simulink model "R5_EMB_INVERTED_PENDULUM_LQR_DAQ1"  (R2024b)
settings: Solver=FixedStepDiscrete  StartTime=0.0  StopTime=S  FixedStep=T  RelTol=1e-3  EnableMultiTasking=on
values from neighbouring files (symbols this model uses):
  A_obs_d = Ad - Ld*C_meas    [R5_EMB_INVERTED_PENDULUM_LQR_DAQ1_script.m]
  B_obs_d = [Bd, Ld]    [R5_EMB_INVERTED_PENDULUM_LQR_DAQ1_script.m]
  C_obs_d = eye(4)    [R5_EMB_INVERTED_PENDULUM_LQR_DAQ1_script.m]
  D_obs_d = zeros(4, 1 + size(C_meas,1))    [R5_EMB_INVERTED_PENDULUM_LQR_DAQ1_script.m]
  Kd = dlqr(Ad, Bd, Q, R)    [R5_EMB_INVERTED_PENDULUM_LQR_DAQ1_script.m]
  Kt = Kt*motor_eff    (= 0.0273)    [R5_EMB_INVERTED_PENDULUM_LQR_DAQ1_script.m]
  r = 0.01    [R5_EMB_INVERTED_PENDULUM_LQR_DAQ1_script.m]
  T = 0.001    [R5_EMB_INVERTED_PENDULUM_LQR_DAQ1_script.m]
undefined symbols (not defined in the file or in its folder): Serial_Port, Standard_Devices
libraries: easyio x6, simulink x5

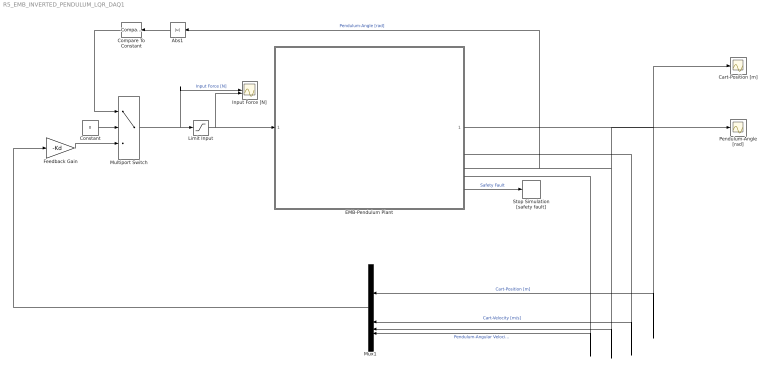
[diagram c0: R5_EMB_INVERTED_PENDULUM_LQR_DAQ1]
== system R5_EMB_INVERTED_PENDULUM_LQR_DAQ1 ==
  Abs1 : Abs
  Cart-Position [m] : Scope
  Compare To Constant : simulink/Logic and Bit Operations/Compare To Constant  relop=<=  const=0.2  OutDataTypeStr=boolean
  Constant : Constant  Value=0
  EMB-Pendulum Plant : Subsystem
  Feedback Gain : Gain  Gain=-Kd  Multiplication=Matrix(K*u)
  Input Force [N] : Scope  NumInputPorts=2
  Limit Input : Saturate  UpperLimit=10  LowerLimit=-10
  Multiport Switch : MultiPortSwitch  DataPortOrder=Zero-based contiguous  Inputs=2  zeroidx=on
  Mux1 : Mux
  Pendulum-Angle [rad] : Scope
  Stop Simulation [safety fault] : Stop
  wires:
  EMB-Pendulum Plant/5(Out5) -> Stop Simulation [safety fault]/1  "Safety Fault"
  Compare To Constant/1 -> Multiport Switch/1
  Multiport Switch/1 -> Input Force [N]/1, Limit Input/1  "Input Force [N]"
  Feedback Gain/1 -> Multiport Switch/3
  Abs1/1 -> Compare To Constant/1
  Limit Input/1 -> EMB-Pendulum Plant/1(In1), Input Force [N]/2
  Constant/1 -> Multiport Switch/2
  Mux1/1 -> Feedback Gain/1
  EMB-Pendulum Plant/4(Out4) -> Mux1/4  "Pendulum-Angular Velocity [rad/s]"
  EMB-Pendulum Plant/1(Out1) -> Cart-Position [m]/1, Mux1/1  "Cart-Position [m]"
  EMB-Pendulum Plant/3(Out3) -> Abs1/1, Mux1/3, Pendulum-Angle [rad]/1  "Pendulum-Angle [rad]"
  EMB-Pendulum Plant/2(Out2) -> Mux1/2  "Cart-Velocity [m/s]"

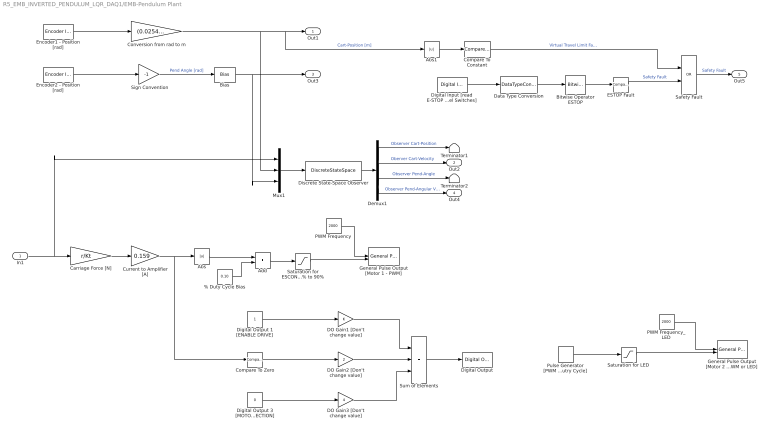
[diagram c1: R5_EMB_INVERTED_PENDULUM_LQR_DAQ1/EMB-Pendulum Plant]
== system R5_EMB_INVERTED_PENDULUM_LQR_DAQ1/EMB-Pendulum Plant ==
  In1 : Inport
  " Sign Convention" : Gain  Gain=-1
  % Duty Cycle Bias : Constant  Value=0.10  SampleTime=T
  Abs : Abs
  Abs1 : Abs
  Add : Sum
  Bias : Bias  Bias=-pi
  Bitwise Operator ESTOP : simulink/Logic and Bit Operations/Bitwise Operator  logicop=AND  UseBitMask=on  BitMask=8  BitMaskRealWorld=Real World Value
  Carriage Force [N] : Gain  Gain=r/Kt
  Compare To Constant : simulink/Logic and Bit Operations/Compare To Constant  relop=>=  const=0.035  OutDataTypeStr=boolean
  Compare To Zero : simulink/Logic and Bit Operations/Compare To Zero  relop=>=  OutDataTypeStr=boolean
  Conversion from rad to m : Gain  Gain=(0.0254)/(2*pi)
  Current to Amplifier [A] : Gain  Gain=0.159
  DO Gain1 [Don't change value] : Gain
  DO Gain2 [Don't change value] : Gain  Gain=2
  DO Gain3 [Don't change value] : Gain  Gain=4
  Data Type Conversion : DataTypeConversion  OutDataTypeStr=uint8  RndMeth=Nearest
  Demux1 : Demux
  Digital Input [read E-STOP and End of Travel Switches] : easyio/Digital Input  SampleTime=T  MaxMissedTicks=10  ShowMissedTicks=0  YieldWhenWaiting=0  DrvName=Standard_Devices/Serial_Port  DrvAddress=6  DrvOptions=[460800 8 0 0 0 0 0 0]  PacketSize=8  DataTypes='double'  ShowReady=0  ShowError=0  PacketID=1  ByteOrder=1  ShowTimestamp=0  CfgPrm=D0  PrmCfg=18  ResVar=0  VarRes=0  d7=off  d6=off  d5=off  d4=on  d3=on  d2=off  d1=off  d0=off
  Digital Output : easyio/Digital Output  SampleTime=T  MaxMissedTicks=10  ShowMissedTicks=0  YieldWhenWaiting=0  DrvName=Standard_Devices/Serial_Port  DrvAddress=6  DrvOptions=[460800 8 0 0 0 0 0 0]  PacketSize=8  DataTypes='double'  ShowReady=0  ShowError=0  PacketID=1  ByteOrder=1  InitialValue=0  FinalValue=0  CfgPrm=G0  PrmCfg=F8  ResVar=0  VarRes=0  d7=off  d6=off  d5=off  d4=off  d3=off  d2=on  d1=on  d0=on
  Digital Output 1 [ENABLE DRIVE] : Constant  SampleTime=T
  Digital Output 3 [MOTOR 2 DIRECTION] : Constant  Value=0  SampleTime=T
  Discrete State-Space Observer : DiscreteStateSpace  A=A_obs_d  B=B_obs_d  C=C_obs_d  D=D_obs_d  InitialCondition=[0 0 0 0]  SampleTime=T
  ESTOP Fault : simulink/Logic and Bit Operations/Compare To Constant  relop=~=  const=8  OutDataTypeStr=boolean
  Encoder1 - Position [rad] : easyio/Encoder Input  SampleTime=T  MaxMissedTicks=10  ShowMissedTicks=0  YieldWhenWaiting=0  DrvName=Standard_Devices/Serial_Port  DrvAddress=6  DrvOptions=[460800 8 0 0 0 0 0 0]  PacketSize=8  DataTypes='double'  ShowReady=0  ShowError=0  PacketID=1  ByteOrder=1  ShowTimestamp=0  CfgPrm=E0  PrmCfg=position  ResVar=0  VarRes=2000
  Encoder2 - Position [rad] : easyio/Encoder Input  SampleTime=T  MaxMissedTicks=10  ShowMissedTicks=0  YieldWhenWaiting=0  DrvName=Standard_Devices/Serial_Port  DrvAddress=6  DrvOptions=[460800 8 0 0 0 0 0 0]  PacketSize=8  DataTypes='double'  ShowReady=0  ShowError=0  PacketID=1  ByteOrder=1  ShowTimestamp=0  CfgPrm=E1  PrmCfg=position  ResVar=0  VarRes=2048
  General Pulse Output [Motor 1 - PWM] : easyio/General Pulse Output  SampleTime=T  MaxMissedTicks=10  ShowMissedTicks=0  YieldWhenWaiting=0  DrvName=Standard_Devices/Serial_Port  DrvAddress=6  DrvOptions=[460800 8 0 0 0 0 0 0]  PacketSize=16  DataTypes={'double','double'}  ShowReady=0  ShowError=0  PacketID=1  ByteOrder=1  InitialValue=[0 0]  FinalValue=[0 0]  CfgPrm=N0  PrmCfg=frequency and duty  ResVar=449.8360 Hz - 115156.25 Hz  VarRes=64
  General Pulse Output [Motor 2 - PWM or LED] : easyio/General Pulse Output  SampleTime=T  MaxMissedTicks=10  ShowMissedTicks=0  YieldWhenWaiting=0  DrvName=Standard_Devices/Serial_Port  DrvAddress=6  DrvOptions=[460800 8 0 0 0 0 0 0]  PacketSize=16  DataTypes={'double','double'}  ShowReady=0  ShowError=0  PacketID=1  ByteOrder=1  InitialValue=[0 0]  FinalValue=[0 0]  CfgPrm=N1  PrmCfg=frequency and duty  ResVar=449.8360 Hz - 115156.25 Hz  VarRes=64
  Mux1 : Mux  Inputs=3
  PWM Frequency : Constant  Value=2000  SampleTime=T
  PWM Frequency_LED : Constant  Value=2000  SampleTime=T
  Pulse Generator [PWM % Dutry Cycle] : DiscretePulseGenerator  PulseType=Time based  Period=0.4  PulseWidth=50
  Safety Fault : Logic  Operator=OR  AllPortsSameDT=off  OutDataTypeStr=boolean
  Saturation for ESCON 10% to 90% : Saturate  UpperLimit=0.9  LowerLimit=0.1
  Saturation for LED : Saturate  UpperLimit=1  LowerLimit=0
  Sum of Elements : Sum  Inputs=+++
  Terminator1 : Terminator
  Terminator2 : Terminator
  Out1 : Outport
  Out2 : Outport  Port=2
  Out3 : Outport  Port=3
  Out4 : Outport  Port=4
  Out5 : Outport  Port=5
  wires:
  % Duty Cycle Bias/1 -> Add/2
  Current to Amplifier [A]/1 -> Abs/1, Compare To Zero/1
  Saturation for ESCON 10% to 90%/1 -> General Pulse Output [Motor 1 - PWM]/2
  DO Gain2 [Don't change value]/1 -> Sum of Elements/2
  PWM Frequency/1 -> General Pulse Output [Motor 1 - PWM]/1
  DO Gain1 [Don't change value]/1 -> Sum of Elements/1
  Digital Output 1 [ENABLE DRIVE]/1 -> DO Gain1 [Don't change value]/1
  Saturation for LED/1 -> General Pulse Output [Motor 2 - PWM or LED]/2
  PWM Frequency_LED/1 -> General Pulse Output [Motor 2 - PWM or LED]/1
  Carriage Force [N]/1 -> Current to Amplifier [A]/1
  Pulse Generator [PWM % Dutry Cycle]/1 -> Saturation for LED/1
  Encoder1 - Position [rad]/1 -> Conversion from rad to m/1
  Sum of Elements/1 -> Digital Output/1
  Add/1 -> Saturation for ESCON 10% to 90%/1
  Compare To Zero/1 -> DO Gain2 [Don't change value]/1
  Abs/1 -> Add/1
  Digital Output 3 [MOTOR 2 DIRECTION]/1 -> DO Gain3 [Don't change value]/1
  DO Gain3 [Don't change value]/1 -> Sum of Elements/3
  Bitwise Operator ESTOP/1 -> ESTOP Fault/1
  Data Type Conversion/1 -> Bitwise Operator ESTOP/1
  Digital Input [read E-STOP and End of Travel Switches]/1 -> Data Type Conversion/1
  Abs1/1 -> Compare To Constant/1
  Compare To Constant/1 -> Safety Fault/1  "Virtual Travel Limit Fault"
  Safety Fault/1 -> Out5/1  "Safety Fault"
  ESTOP Fault/1 -> Safety Fault/2  "Safety Fault"
  " Sign Convention"/1 -> Bias/1  "Pend Angle [rad]"
  Encoder2 - Position [rad]/1 -> " Sign Convention"/1
  Demux1/2 -> Out2/1  "Oberver Cart-Velocity"
  Discrete State-Space Observer/1 -> Demux1/1
  Demux1/4 -> Out4/1  "Observer Pend-Angular Velocity"
  Demux1/3 -> Terminator2/1  "Observer Pend-Angle"
  Conversion from rad to m/1 -> Abs1/1, Out1/1, Mux1/2  "Cart-Position [m]"
  Bias/1 -> Out3/1, Mux1/3
  In1/1 -> Mux1/1, Carriage Force [N]/1
  Mux1/1 -> Discrete State-Space Observer/1
  Demux1/1 -> Terminator1/1  "Observer Cart-Position"
